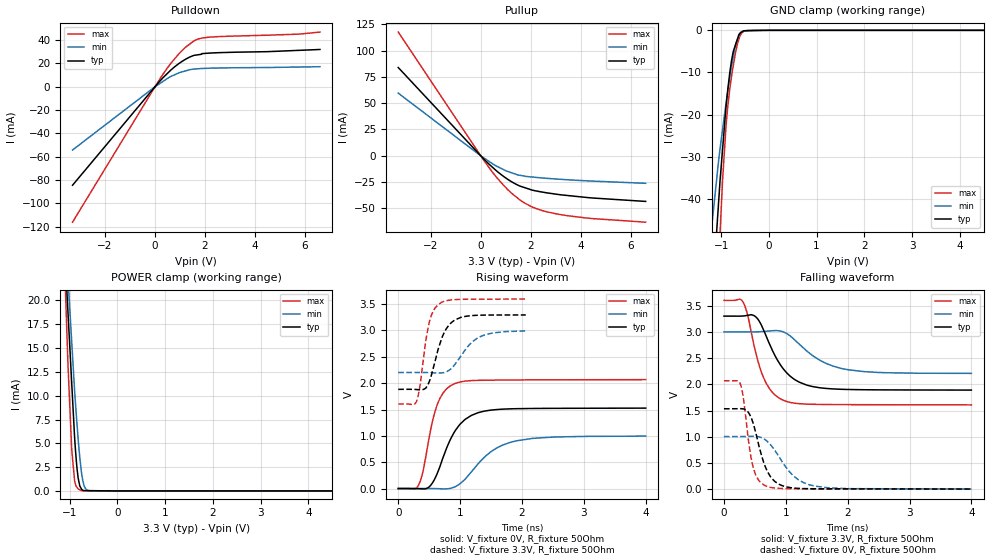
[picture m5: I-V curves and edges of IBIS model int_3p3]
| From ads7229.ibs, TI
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|   int_3p3 Model
[Model]   int_3p3
Model_type   I/O
Polarity   Non-Inverting
Enable   Active-Low
Vinl = 1.155
Vinh = 2.145
Vmeas = 1.65
Vref = 1.65
Cref = 30pF
Rref = 50
|   typ   min   max
|   (nom PVT)   (Fast PVT)   (slow PVT)
|C_comp from frequency sweep method(F=50MHz)
C_comp   5.061e-12   4.100e-12   5.975e-12
|OFF state: BUFFER IN HIGH IMPEDANCE
|C_comp   5.061e-12   4.100e-12   5.975e-12
|ON state : BUFFER OUTPUT TURNED HIGH
|C_comp   5.474e-12   4.490e-12   6.450e-12
|C_comp from LC tank measurement(L=1nH)
|ON state : BUFFER OUTPUT TURNED HIGH
|Resonant Frequency(Hz)   2.450e+09   2.630e+09   2.340e+09
|C_comp   4.224e-12   3.666e-12   4.631e-12
|OFF state: BUFFER IN HIGH IMPEDANCE
|Resonant Frequency   2.550e+09   2.800e+09   2.390e+09
|C_comp   3.899e-12   3.234e-12   4.439e-12
| Where nom  PVT is Nominal Process,  3.3V,  28C
|   Fast PVT is Strong Process,   3.6V,  -40C
|   Slow PVT is Weak Process,   3V,  88C
[Model Spec]
|Subparameter   typ   min   max
Vinh   2.145   1.95   2.34
Vinl   1.155   1.05   1.26
[Voltage Range]   3.3   3   3.6
|Ambient Temperature   25   85   -40
|Junction Temperature
[Temperature Range]   28   88   -40
[Pullup Reference]   3.3   3   3.6
[Pulldown Reference]   0   0   0
[Power Clamp Reference]   3.3   3   3.6
[GND Clamp Reference]   0   0   0
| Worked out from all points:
|   slope of the pulldown table from 0 to 0.495 V, typ, clamps not added: 43.3 ohm
|   slope of the pullup table from 0 to 0.495 V, typ, clamps not added: 43.4 ohm
|   GND clamp passes 1 mA (typ) near -0.62 V on its own axis
|   POWER clamp passes 1 mA (typ) near -0.81 V on its own axis
|   falling waveform, V_fixture 3.3V, R_fixture 50Ohm: 20-80 % time 409ps typ, 573ps min, 285ps max; typ from 3.3 V to 1.89 V
|   rising waveform, V_fixture 0V, R_fixture 50Ohm: 20-80 % time 363ps typ, 541ps min, 237ps max; typ from 0 V to 1.53 V
|   rising waveform, V_fixture 3.3V, R_fixture 50Ohm: 20-80 % time 228ps typ, 335ps min, 154ps max; typ from 1.88 V to 3.29 V
|   falling waveform, V_fixture 0V, R_fixture 50Ohm: 20-80 % time 237ps typ, 394ps min, 151ps max; typ from 1.53 V to 0.006 V
[Pulldown]
|   Voltage   I(typ)   I(min)   I(max)
-3.3V     -84.5mA    -54.28mA   -116.2mA
172.8mV   4.321mA    2.494mA    5.996mA
648mV     14.59mA    8.972mA    20.48mA
939.6mV   19.67mA    11.76mA    27.86mA
1.246V    23.91mA    13.75mA    34.31mA
1.57V     26.96mA    15.2mA     39.49mA
1.811V    27.73mA    15.59mA    41.49mA
2.012V    28.63mA    15.79mA    42.21mA
5.774V    31.25mA    16.94mA    45.18mA
6.6V      31.99mA    17.21mA    46.91mA
[GND Clamp]
|   Voltage   I(typ)   I(min)   I(max)
-3.3V     -515.1mA   -360.9mA   -728.9mA
-1.236V   -72.97mA   -50.81mA   -106.6mA
-1.185V   -63.28mA   -45.24mA   -92.2mA
-1.059V   -41.88mA   -31.6mA    -56.9mA
-1.023V   -35.76mA   -28.13mA   -48.27mA
-896.4mV  -18.01mA   -17.25mA   -22.62mA
-820.8mV  -10.27mA   -11.41mA   -14.07mA
-745.8mV  -5.02mA    -6.286mA   -8.385mA
-696mV    -3.367mA   -3.336mA   -5.168mA
-612mV    -861uA     -747uA     -1.512mA
-537mV    -199uA     -155.1uA   -329.7uA
6.6V      0A         0A         0A
[Pullup]
|   Voltage   I(typ)   I(min)   I(max)
-3.3V     83.87mA    59.52mA    117.5mA
172.8mV   -4.243mA   -2.787mA   -6.008mA
583.2mV   -13.3mA    -9.192mA   -18.99mA
939.6mV   -20.06mA   -13.5mA    -28.71mA
1.246V    -24.85mA   -16.26mA   -35.81mA
1.588V    -28.94mA   -18.64mA   -42.32mA
2.167V    -33.2mA    -20.45mA   -49.72mA
3.089V    -36.75mA   -22.21mA   -55.5mA
4.496V    -40.17mA   -24.1mA    -59.74mA
6.6V      -43.38mA   -26.18mA   -63.12mA
[POWER Clamp]
|   Voltage   I(typ)   I(min)   I(max)
-3.3V     177.2mA    159.9mA    202.3mA
-1.451V   64.21mA    57.65mA    74.34mA
-1.053V   20.33mA    23.74mA    15.72mA
-1.033V   18.48mA    22.08mA    12.9mA
-957.6mV  11.31mA    15.64mA    4.341mA
-896.4mV  5.542mA    10.44mA    1.014mA
-858mV    2.968mA    7.716mA    450.9uA
-825mV    1.431mA    5.571mA    220.1uA
-756mV    227.7uA    2.041mA    37.91uA
-696mV    34.33uA    508.2uA    6.822uA
-591mV    29.13uA    21.79uA    1.713uA
6.6V      0A         0A         0A
[Ramp]
R_load = 50
|   typ   min   max
dV/dt_r   0.915778/3.62758e-10   0.596977/5.36857e-10   1.24016/2.36268e-10
dV/dt_f   0.845614/4.08311e-10   0.474731/5.69099e-10   1.19492/2.84282e-10
[Falling Waveform]
V_fixture = 3.3V
V_fixture_min = 3V
V_fixture_max = 3.6V
R_fixture = 50Ohm
|   Time   V(typ)   V(min)   V(max)
0s        3.3V       3V         3.6V
307ps     3.302V     3V         3.572V
387ps     3.316V     2.999V     3.3V
485ps     3.31V      3V         2.75V
632ps     3.058V     3.007V     2.152V
777ps     2.663V     3.021V     1.857V
967ps     2.284V     2.996V     1.693V
1.332ns   1.988V     2.643V     1.624V
1.92ns    1.905V     2.298V     1.614V
3.999ns   1.891V     2.209V     1.608V
[Rising Waveform]
V_fixture = 0V
V_fixture_min = 0V
V_fixture_max = 0V
R_fixture = 50Ohm
|   Time   V(typ)   V(min)   V(max)
0s        1.151nV    1.335nV    1.032nV
325ps     -1.544mV   251.8uV    57.18mV
408ps     -6.891mV   420.2uV    369.6mV
495ps     27.04mV    274.4uV    939mV
621ps     260.7mV    -1.879mV   1.56V
900ps     1.058V     24.56mV    1.984V
1.184ns   1.389V     318mV      2.049V
1.494ns   1.488V     695mV      2.057V
1.83ns    1.513V     882.7mV    2.061V
3.999ns   1.526V     995mV      2.067V
[Rising Waveform]
V_fixture = 3.3V
V_fixture_min = 3V
V_fixture_max = 3.6V
R_fixture = 50Ohm
|   Time   V(typ)   V(min)   V(max)
0s        1.883V     2.203V     1.605V
296ps     1.879V     2.203V     1.654V
355ps     1.874V     2.203V     1.98V
436ps     1.899V     2.202V     2.727V
494ps     2.008V     2.2V       3.114V
648ps     2.655V     2.192V     3.493V
800ps     3.072V     2.229V     3.571V
1.01ns    3.248V     2.51V      3.591V
1.333ns   3.291V     2.887V     3.594V
2.061ns   3.295V     2.992V     3.596V
[Falling Waveform]
V_fixture = 0V
V_fixture_min = 0V
V_fixture_max = 0V
R_fixture = 50Ohm
|   Time   V(typ)   V(min)   V(max)
0s        1.534V     1.005V     2.068V
261ps     1.537V     1.005V     2.021V
311ps     1.533V     1.006V     1.763V
402ps     1.452V     1.008V     880.8mV
467ps     1.277V     1.01V      447.9mV
677ps     406mV      936.9mV    64.54mV
943ps     69.42mV    520.3mV    15.25mV
1.194ns   18.61mV    189.8mV    9.678mV
1.462ns   10.81mV    63.1mV     8.258mV
3.999ns   5.708mV    6.112mV    3.131mV
